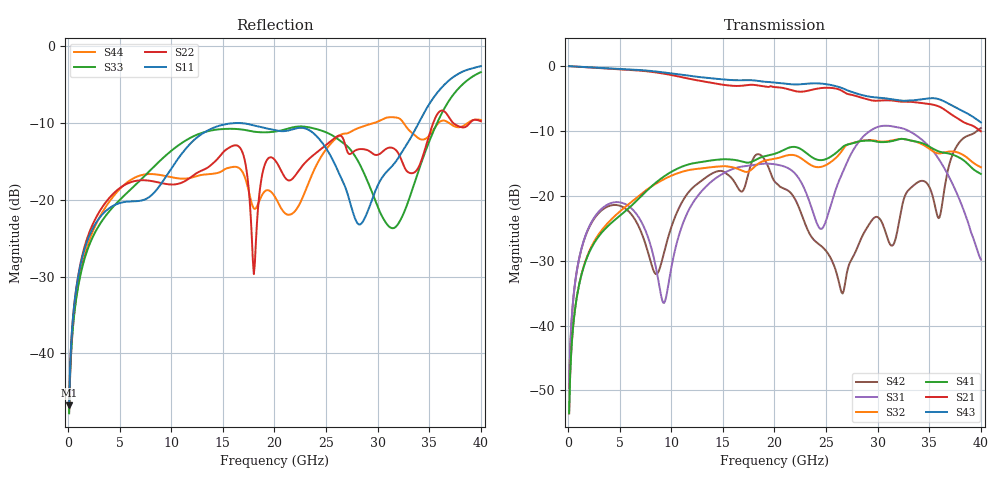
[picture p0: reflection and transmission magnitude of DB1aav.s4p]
! ADC12DJ2700AAV, ADC12DJ3200AAV, ADC08DJ3200AAV
! 144 pin AAV package
! Texas Instruments 4/21/2021
! Single-ended  S-parameters
! PORT#  PORT_NAME  NET_NAME
! PORT1:  DAxN.DIEBUMP DAxN
! PORT2:  DAxN.BGA  DAxN
! PORT3:  DAxP.DIEBUMP DAxP
! PORT4:  DAxP.BGA  DAxP
! Touchstone Ver. 1.0
! Number of ports is 4
# Hz	S	MA	R	50.000000
! SCATTERING PARAMETERS  :
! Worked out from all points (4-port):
!   400 points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, 100 MHz to 40 GHz, reference 50 ohm
!   strongest paths, dB at 100 MHz, 10.1 GHz, 20.1 GHz, 30.1 GHz, 40 GHz:
!     S43: 0.0, -1.1, -2.6, -4.9, -8.7
!     S21: 0.0, -1.4, -3.3, -5.3, -10.1
!     S41: -53.5, -16.2, -13.5, -11.7, -16.6
!     S32: -53.5, -16.8, -14.3, -11.6, -15.6
!     S31: -49.6, -30.3, -15.2, -9.3, -29.8
!     S42: -49.6, -24.4, -17.9, -23.4, -9.6
!   lowest |S11| = -46.8 dB at 100 MHz (marker M1), VSWR 1.01, Z = 50.2 + j0.414 ohm
!   |S11| at or under -10 dB: start of sweep to 16.25 GHz; 16.64 GHz to 33.96 GHz (17.32 GHz wide, 68.5 % of centre)
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1e8  0.004568 64.5  0.9978 -1.5  0.00332 84.8  0.002109 -97.2
     0.9978 -1.5  0.00457 63.8  0.002109 -97.1  0.003317 84.6
     0.00332 84.8  0.002109 -97.1  0.004062 63.4  0.9979 -1.4
     0.002109 -97.2  0.003317 84.6  0.9979 -1.4  0.004077 62.2
2.9e9  0.07406 45.3  0.966 -40.7  0.07437 42.5  0.04791 -146.9
       0.966 -40.7  0.08082 22.8  0.04963 -145.7  0.07268 39.3
       0.07437 42.5  0.04963 -145.7  0.06634 57.3  0.9699 -38.6
       0.04791 -146.9  0.07268 39.3  0.9699 -38.6  0.07367 16.6
1e10  0.1598 29.2  0.853 -137.8  0.02787 79.2  0.153 113.8
      0.853 -137.8  0.1258 -72.8  0.1429 108.5  0.05725 62.4
      0.02787 79.2  0.1429 108.5  0.2086 24.9  0.8784 -130.2
      0.153 113.8  0.05725 62.4  0.8784 -130.2  0.1404 -92.6
2.05e10  0.2806 -68.9  0.6838 92.7  0.1721 -5.7  0.2179 -45.8
         0.6838 92.7  0.1618 173.8  0.1969 -40.8  0.1182 -78.6
         0.1721 -5.7  0.1969 -40.8  0.2816 -53.4  0.7409 102.1
         0.2179 -45.8  0.1182 -78.6  0.7409 102.1  0.09146 174.3
2.66e10  0.1326 -162.5  0.6397 10.1  0.1512 114.5  0.2374 -128.8
         0.6397 10.1  0.2543 -31.4  0.226 -109.9  0.01768 -94.4
         0.1512 114.5  0.226 -109.9  0.2359 -117.6  0.6739 20.8
         0.2374 -128.8  0.01768 -94.4  0.6739 20.8  0.2686 -47.4
3.16e10  0.172 8.1  0.5401 -50.4  0.3411 16.9  0.2664 143.5
         0.5401 -50.4  0.2152 -72.4  0.269 160.0  0.04327 106.9
         0.3411 16.9  0.269 160.0  0.06561 148.2  0.5514 -36.7
         0.2664 143.5  0.04327 106.9  0.5514 -36.7  0.345 -99.8
4e10  0.7426 -79.1  0.3142 -168.4  0.03225 -37.4  0.1474 -5.3
      0.3142 -168.4  0.3252 -89.9  0.1659 19.3  0.3328 78.2
      0.03225 -37.4  0.1659 19.3  0.6791 -45.9  0.3681 -154.3
      0.1474 -5.3  0.3328 78.2  0.3681 -154.3  0.3317 -120.5
